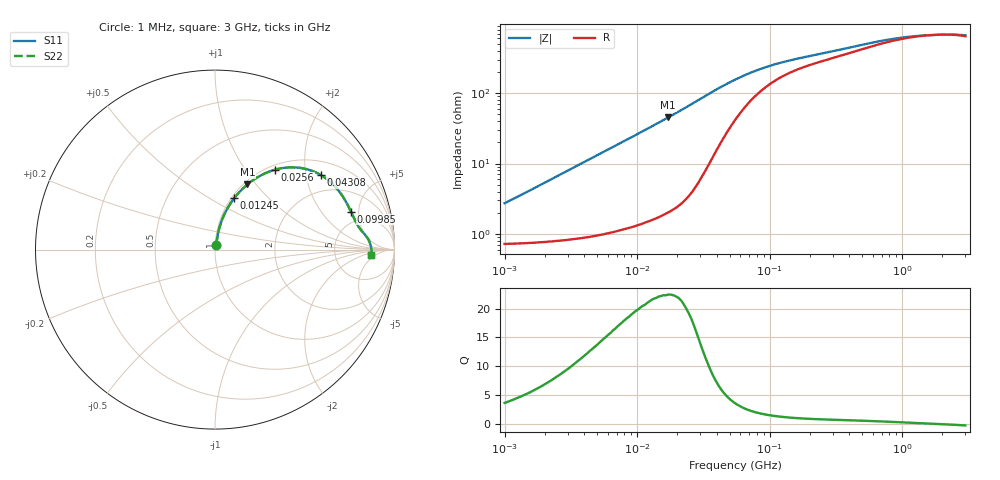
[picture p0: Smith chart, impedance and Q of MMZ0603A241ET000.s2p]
! S-Parameter Data Generated by TDK Corporation
! Copyright(C) 2025 TDK Corporation.
! All Rights Reserved.
! TDK P/N: MMZ0603A241ET000 (Chip Bead)
! Property: |Z|=240ohm at 100MHz
! Size(LxWxT): 0.6x0.3x0.3mm
! Model Type: s2p (Touchstone File Format Version 1.0)
! Frequency: DC=Yes Start=1MHz Stop=3000MHz 202points Log-sweep
! Model Generated on Feb. 6, 2025
! Terms and conditions regarding TDK Simulation Models:
! 1)This simulation model is being provided solely for informational
!  purposes. Please refer to the specifications of the products in
!  terms of detailed characteristics of such products.
! 2)In no event shall TDK Corporation of any of its subsidiaries be
!  liable for any loss or damage arising, directly or indirectly,
!  from any information contained in this simulation model, including,
!  but not limited to loss or damages arising from any inaccuracies,
!  omissions or errors in connection with such information.
! 3)Any and all copyrights on this simulation model are owned by
!  TDK Corporation.  Duplication or redistribution of this simulation
!  model without prior written permission from TDK Corporation
!  is prohibited.
! 4)This simulation model is subject to any modification or change
!  without any prior notice.
! 5)Neither TDK Corporation nor any of its subsidiaries shall make any
!  warranty, express or implied, including but not limited to the
!  correctness, implied warranties of merchantability and fitness for
!  a particular purpose with respect to this simulation models.
! 6)The use of this simulation model shall be deemed to have consented
!  to the terms and conditions hereof.
! Port Assignments:
!  1 ---@@@--- 2
! Applicable Conditions:
!  Temperature = 25 degC
!  DC Bias Current = 0 A
!  Small Signal Operation
# Hz S MA R 50
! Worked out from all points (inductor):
!   201 points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, 1 MHz to 3 GHz, reference 50 ohm
!   read as one part in series: L = 419 nH near 1.041 MHz
!   highest Q = 22.3 at 17.15 MHz (marker M1), where L = 419 nH
!   self-resonance near 1.927 GHz
!   S11 on the Smith chart (normalised r, x): 1 MHz: 1.01, +0.05; 12.45 MHz: 1.03, +0.65; 25.6 MHz: 1.08, +1.39; 43.08 MHz: 1.41, +2.43; 99.85 MHz: 3.68, +4.09; 3 GHz: 14, -3
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1000000  0.02712 73.2  0.9925 -1.5  0.9925 -1.5  0.02712 73.2
2139570  0.05628 78.9  0.9907 -3.2  0.9907 -3.2  0.05628 78.9
3900413  0.1011 79.3  0.9862 -5.8  0.9862 -5.8  0.1011 79.3
7703107  0.1953 75.5  0.9697 -11.2  0.9697 -11.2  0.1953 75.5
1.245355e7  0.3057 69.5  0.9379 -17.8  0.9379 -17.8  0.3057 69.5
1.461624e7  0.3529 66.8  0.9199 -20.6  0.9199 -20.6  0.3529 66.8
1.71545e7  0.4055 63.5  0.8962 -23.9  0.8962 -23.9  0.4055 63.5
2.095589e7  0.4787 58.8  0.8562 -28.6  0.8562 -28.6  0.4787 58.8
2.559965e7  0.5571 53.1  0.8006 -33.8  0.8006 -33.8  0.5571 53.1
3.254976e7  0.6464 45.0  0.7098 -40.1  0.7098 -40.1  0.6464 45.0
3.670325e7  0.6834 40.7  0.6569 -42.8  0.6569 -42.8  0.6834 40.7
4.307715e7  0.7207 35.2  0.5847 -45.3  0.5847 -45.3  0.7207 35.2
5.477226e7  0.7549 27.9  0.4847 -46.7  0.4847 -46.7  0.7549 27.9
6.964249e7  0.7726 21.9  0.404 -45.5  0.404 -45.5  0.7726 21.9
9.984923e7  0.7868 15.6  0.3217 -41.2  0.3217 -41.2  0.7868 15.6
1.431579e8  0.7977 11.6  0.2713 -36.3  0.2713 -36.3  0.7977 11.6
2.136344e8  0.8113 8.8  0.2342 -32.1  0.2342 -32.1  0.8113 8.8
8.005644e8  0.8607 3.1  0.148 -18.2  0.148 -18.2  0.8607 3.1
1.147801e9  0.8672 1.8  0.1358 -11.3  0.1358 -11.3  0.8672 1.8
1.581072e9  0.8705 0.6  0.13 -4.3  0.13 -4.3  0.8705 0.6
2.266846e9  0.8728 -0.6  0.1275 4.0  0.1275 4.0  0.8728 -0.6
3e9  0.8723 -1.8  0.1311 12.1  0.1311 12.1  0.8723 -1.8
